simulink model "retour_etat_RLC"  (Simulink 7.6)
settings: Solver=ode23tb  StartTime=0.0  StopTime=0.25  RelTol=1e-3
InitFcn:
  | % valeurs de R, L et C
  | R=3.3;
  | L=100e-3;
  | C=1e-3;
  | 
  | % coefficients du retour d'état
  | f1=-0.1568;
  | f2= -0.6909;
StopFcn:
  | close all, clc
  | load u_bo_u_bf.mat
  | subplot 211
  | plotyy(x(1,:),x(2,:),x(1,:),x(3,:))
  | xlabel('temps')
  | title('Tension u en boucle ouverte et fermée')
  | grid
  | 
  | subplot 212
  | load i_bo_i_bf.mat
  | plotyy(y(1,:),y(2,:),y(1,:),y(3,:))
  | grid
  | title('Courant i en boucle ouverte et fermée')
  | delete *.mat
undefined symbols (not defined in the file or in its folder): T
libraries: powerlib x14

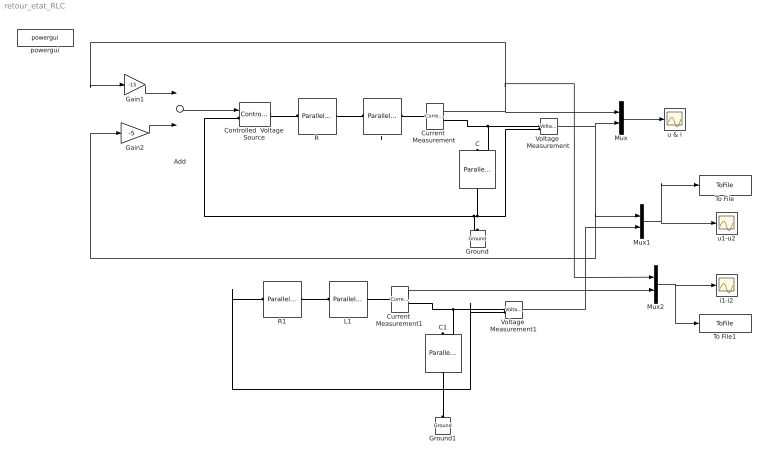
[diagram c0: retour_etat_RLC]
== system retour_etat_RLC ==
  Add : Sum
  C : powerlib/Elements/Parallel RLC Branch  DialogController=POWERSYS.PowerSysDialog  PhysicalDomain=powersysdomain  SubClassName=unknown  LeftPortType=p1  RightPortType=p1  LConnTagsString=a  RConnTagsString=__new0  BranchType=C  Resistance=1e-3  Inductance=1e-3  SetiL0=off  InitialCurrent=0  Capacitance=C  Setx0=on  InitialVoltage=0.1  Measurements=None
  C1 : powerlib/Elements/Parallel RLC Branch  DialogController=POWERSYS.PowerSysDialog  PhysicalDomain=powersysdomain  SubClassName=unknown  LeftPortType=p1  RightPortType=p1  LConnTagsString=a  RConnTagsString=__new0  BranchType=C  Resistance=1e-3  Inductance=1e-3  SetiL0=off  InitialCurrent=0  Capacitance=C  Setx0=on  InitialVoltage=0.1  Measurements=None
  Controlled  Voltage Source : powerlib/Electrical Sources/Controlled Voltage Source  DialogController=POWERSYS.PowerSysDialog  SystemSampleTime=-1  Initialize=on  Source_Type=AC  Amplitude=0  Phase=0  Frequency=0  Measurements=None
  Current  Measurement : powerlib/Measurements/Current Measurement  DialogController=POWERSYS.PowerSysDialog  SystemSampleTime=-1  PhasorSimulation=off  OutputType=Complex  PSBequivalent=0
  Current  Measurement1 : powerlib/Measurements/Current Measurement  DialogController=POWERSYS.PowerSysDialog  SystemSampleTime=-1  PhasorSimulation=off  OutputType=Complex  PSBequivalent=0
  Gain1 : Gain  Gain=-15
  Gain2 : Gain  Gain=-5
  Ground : powerlib/Elements/Ground  DialogController=POWERSYS.PowerSysDialog  PhysicalDomain=powersysdomain  SubClassName=unknown  LeftPortType=p1  RightPortType=p1  LConnTagsString=a
  Ground1 : powerlib/Elements/Ground  DialogController=POWERSYS.PowerSysDialog  PhysicalDomain=powersysdomain  SubClassName=unknown  LeftPortType=p1  RightPortType=p1  LConnTagsString=a
  L : powerlib/Elements/Parallel RLC Branch  DialogController=POWERSYS.PowerSysDialog  PhysicalDomain=powersysdomain  SubClassName=unknown  LeftPortType=p1  RightPortType=p1  LConnTagsString=a  RConnTagsString=__new0  BranchType=L  Resistance=1e-3  Inductance=L  SetiL0=on  InitialCurrent=-0.04  Capacitance=1e-6  Setx0=off  InitialVoltage=0  Measurements=None
  L1 : powerlib/Elements/Parallel RLC Branch  DialogController=POWERSYS.PowerSysDialog  PhysicalDomain=powersysdomain  SubClassName=unknown  LeftPortType=p1  RightPortType=p1  LConnTagsString=a  RConnTagsString=__new0  BranchType=L  Resistance=1e-3  Inductance=L  SetiL0=on  InitialCurrent=-0.04  Capacitance=1e-6  Setx0=off  InitialVoltage=0  Measurements=None
  Mux : Mux  Inputs=2
  Mux1 : Mux  Inputs=2
  Mux2 : Mux  Inputs=2
  R : powerlib/Elements/Parallel RLC Branch  DialogController=POWERSYS.PowerSysDialog  PhysicalDomain=powersysdomain  SubClassName=unknown  LeftPortType=p1  RightPortType=p1  LConnTagsString=a  RConnTagsString=__new0  BranchType=R  Resistance=R  Inductance=1e-3  SetiL0=off  InitialCurrent=0  Capacitance=1e-6  Setx0=off  InitialVoltage=0  Measurements=None
  R1 : powerlib/Elements/Parallel RLC Branch  DialogController=POWERSYS.PowerSysDialog  PhysicalDomain=powersysdomain  SubClassName=unknown  LeftPortType=p1  RightPortType=p1  LConnTagsString=a  RConnTagsString=__new0  BranchType=R  Resistance=R  Inductance=1e-3  SetiL0=off  InitialCurrent=0  Capacitance=1e-6  Setx0=off  InitialVoltage=0  Measurements=None
  To File : ToFile  Filename=u_bo_u_bf  MatrixName=x
  To File1 : ToFile  Filename=i_bo_i_bf  MatrixName=y
  Voltage  Measurement : powerlib/Measurements/Voltage Measurement  DialogController=POWERSYS.PowerSysDialog  SystemSampleTime=-1  PhasorSimulation=off  OutputType=Complex  PSBequivalent=0
  Voltage  Measurement1 : powerlib/Measurements/Voltage Measurement  DialogController=POWERSYS.PowerSysDialog  SystemSampleTime=-1  PhasorSimulation=off  OutputType=Complex  PSBequivalent=0
  i1-i2 : Scope
  powergui : powerlib/powergui  Priority=1  SystemSampleTime=-1  SimulationMode=Continuous  SampleTime=T  frequency=60  SPID=off  DisableSnubberDevices=off  DisableRonSwitches=off  DisableVfSwitches=off  SwTol=0  Interpol=off  frequencyindice=0  echomessages=off  HookPort=off  DisplayEquations=off  FunctionMessages=off  EnableUseOfTLC=off  x0status=blocks  RestoreLinks=warning  ResistiveCurrentMeasurement=off  Ylog=off  Xlog=on  ShowGrid=off  save=off  variable=ZData  ZoomFFT=off  StartTime=0.0  cycles=1  DisplayStyle=1  FreqAxis=off  MaxFrequency=1000  frequencyindicesteady=1  display=off  methode=off
  u & i : Scope
  u1-u2 : Scope
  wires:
  Voltage  Measurement/1 -> Mux/2, Mux1/1, Gain2/1
  Current  Measurement/1 -> Mux/1, Gain1/1, Mux2/1
  Mux/1 -> u & i/1
  Gain1/1 -> Add/1
  Gain2/1 -> Add/2
  Voltage  Measurement1/1 -> Mux1/2
  Current  Measurement1/1 -> Mux2/2
  Mux1/1 -> u1-u2/1, To File/1
  Mux2/1 -> i1-i2/1, To File1/1
  Add/1 -> Controlled  Voltage Source/1
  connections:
  R/RConn1 -- L/LConn1
  Voltage  Measurement/LConn1 -- C/LConn1 -- Current  Measurement/RConn1
  C/RConn1 -- Ground/LConn1 -- Controlled  Voltage Source/LConn1 -- Voltage  Measurement/LConn2
  Controlled  Voltage Source/RConn1 -- R/LConn1
  L/RConn1 -- Current  Measurement/LConn1
  Voltage  Measurement1/LConn1 -- Current  Measurement1/RConn1 -- C1/LConn1
  C1/RConn1 -- Ground1/LConn1 -- R1/LConn1 -- Voltage  Measurement1/LConn2
  L1/RConn1 -- Current  Measurement1/LConn1
  R1/RConn1 -- L1/LConn1
